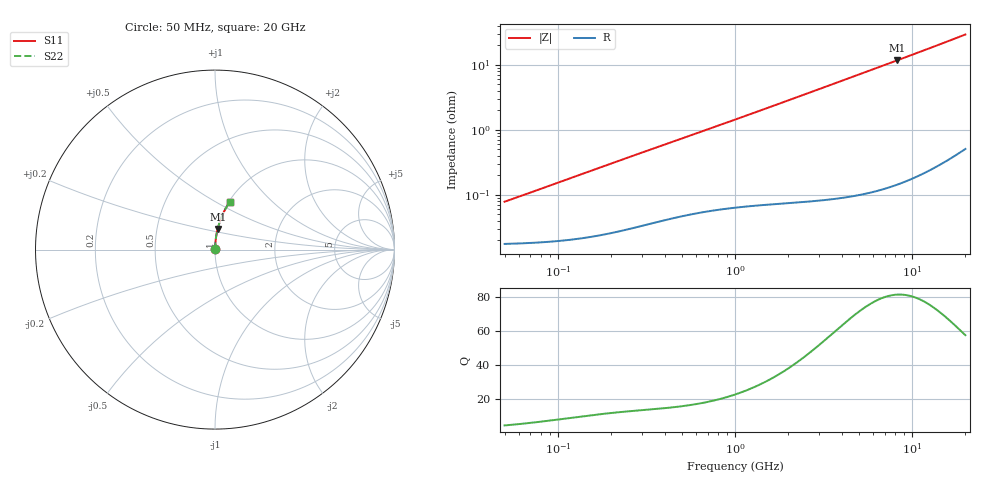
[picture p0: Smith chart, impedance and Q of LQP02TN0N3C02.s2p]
!Murata Part Number: LQP02TN0N3C02
!These Parameters are Measured in Series Mode Connection
!  o--[Z]--o
!Port1  Port2
!  o-------o
!Freq. Start=50[MHz] Stop=20[GHz], 401[Steps]
# Hz S RI R 50
!Freq.(Hz) S11(Real) S11(Imag) S21(Real) S21(Imag) S12(Real) S12(Imag) S22(Real) S22(Imag)
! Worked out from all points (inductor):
!   401 points, 50 MHz to 20 GHz, reference 50 ohm
!   read as one part in series: L = 244 pH near 51.52 MHz
!   highest Q = 81.5 at 8.265 GHz (marker M1), where L = 226 pH
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5e7  0.000177 0.000766  0.9998 -0.000766  0.9998 -0.000766  0.000177 0.000766
5.152053e7  0.000177 0.000789  0.9998 -0.000789  0.9998 -0.000789  0.000177 0.000789
6.07487e7  0.00018 0.00093  0.9998 -0.00093  0.9998 -0.00093  0.00018 0.00093
1.364002e8  0.000219 0.00208  0.9998 -0.00208  0.9998 -0.00208  0.000219 0.00208
2.304068e8  0.000294 0.00347  0.9997 -0.00347  0.9997 -0.00347  0.000294 0.00347
3.721004e8  0.000419 0.00552  0.9996 -0.00552  0.9996 -0.00552  0.000419 0.00552
6.380365e8  0.000619 0.00927  0.9994 -0.00927  0.9994 -0.00927  0.000619 0.00927
1e9  0.00084 0.0143  0.9992 -0.0143  0.9992 -0.0143  0.00084 0.0143
1.714689e9  0.00132 0.0243  0.9987 -0.0243  0.9987 -0.0243  0.00132 0.0243
2.728004e9  0.00229 0.0385  0.9977 -0.0385  0.9977 -0.0385  0.00229 0.0385
3.626126e9  0.00349 0.0511  0.9965 -0.0511  0.9965 -0.0511  0.00349 0.0511
4.677679e9  0.00531 0.0658  0.9947 -0.0658  0.9947 -0.0658  0.00531 0.0658
5.944466e9  0.00812 0.0835  0.9919 -0.0835  0.9919 -0.0835  0.00812 0.0835
7.442007e9  0.0123 0.1042  0.9877 -0.1042  0.9877 -0.1042  0.0123 0.1042
8.264682e9  0.015 0.1155  0.985 -0.1155  0.985 -0.1155  0.015 0.1155
9.457416e9  0.0194 0.1318  0.9806 -0.1318  0.9806 -0.1318  0.0194 0.1318
1.066139e10  0.0244 0.1481  0.9756 -0.1481  0.9756 -0.1481  0.0244 0.1481
1.201863e10  0.0308 0.1663  0.9692 -0.1663  0.9692 -0.1663  0.0308 0.1663
1.354865e10  0.0388 0.1864  0.9612 -0.1864  0.9612 -0.1864  0.0388 0.1864
1.646126e10  0.0567 0.2238  0.9433 -0.2238  0.9433 -0.2238  0.0567 0.2238
1.940974e10  0.0782 0.2601  0.9218 -0.2601  0.9218 -0.2601  0.0782 0.2601
2e10  0.0829 0.2671  0.9171 -0.2671  0.9171 -0.2671  0.0829 0.2671
